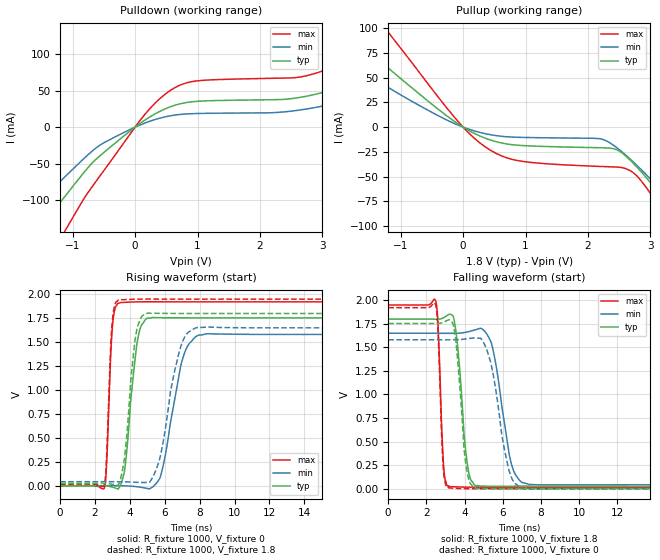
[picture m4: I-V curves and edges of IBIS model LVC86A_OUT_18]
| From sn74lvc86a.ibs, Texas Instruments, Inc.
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[Model]   LVC86A_OUT_18
Model_type  Output
Vref =   0
Rref =   1000
Cref =   30p
Vmeas =   0.9
| variable   typ   min   max
C_comp   6.28pF   4.38pF   8.30pF
| C_pullup   5.89pF   4.38pF   6.79pF
| C_pulldown   6.66pF   4.69pF   8.30pF
[Temperature Range]   40   100   -40
| Ambient temperature   25   85   -40
[Voltage range]   1.8   1.65   1.95
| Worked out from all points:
|   slope of the pulldown table from 0 to 0.27 V, typ, clamps not added: 17.1 ohm
|   slope of the pullup table from 0 to 0.27 V, typ, clamps not added: 29.9 ohm
|   rising waveform, R_fixture 1000, V_fixture 0: 20-80 % time 535ps typ, 904ps min, 249ps max; typ from 0 V to 1.75 V
|   falling waveform, R_fixture 1000, V_fixture 1.8: 20-80 % time 403ps typ, 707ps min, 210ps max; typ from 1.8 V to 0.027 V
|   rising waveform, R_fixture 1000, V_fixture 1.8: 20-80 % time 501ps typ, 925ps min, 244ps max; typ from 0.027 V to 1.8 V
|   falling waveform, R_fixture 1000, V_fixture 0: 20-80 % time 391ps typ, 743ps min, 203ps max; typ from 1.75 V to 0 V
[Pulldown]
| LVC86A_OUT_18
|   Voltage   I(typ)   I(min)   I(max)
-5.5V     -559.1mA   -452.2mA   -710.9mA
-2.18V    -208.5mA   -158.8mA   -285.4mA
-1.865V   -175.2mA   -131.6mA   -244.5mA
-1.48V    -133.9mA   -98.56mA   -193.1mA
-1.07V    -89.31mA   -63.76mA   -134.9mA
70mV      4.491mA    2.617mA    8.125mA
615mV     29.45mA    16.27mA    53.12mA
2.815V    43.69mA    25.92mA    72.1mA
4.325V    93.52mA    64.21mA    142.7mA
5.155V    134.5mA    96.03mA    199.6mA
6.155V    191.3mA    141.3mA    276.1mA
11V       510.2mA    405.2mA    689.3mA
[Pullup]
| LVC86A_OUT_18
|   Voltage   I(typ)   I(min)   I(max)
-5.5V     324.9mA    249.5mA    454.8mA
-2.68V    143.9mA    103mA      216.3mA
-2.015V   104.9mA    73.15mA    161.8mA
-1.32V    66.21mA    44.72mA    105.6mA
360mV     -11.3mA    -6.711mA   -20.18mA
985mV     -18.72mA   -10.42mA   -34.9mA
2.465V    -23.02mA   -20.97mA   -40.36mA
2.785V    -40.46mA   -38.76mA   -49.43mA
3.365V    -85.63mA   -77.45mA   -103.2mA
3.56V     -102.6mA   -91.66mA   -124.4mA
3.775V    -122mA     -107.8mA   -148.7mA
11V       -874.4mA   -739.7mA   -1.068A
[Ramp]
| LVC86A_OUT_18
| variable   typ   min   max
dV/dt_r   1.07/5.81E-10   0.97/9.92E-10   1.17/2.64E-10
dV/dt_f   1.10/4.49E-10   1.00/7.86E-10   1.20/2.28E-10
R_load = 1000
[Rising Waveform]
| LVC86A_OUT_18
R_fixture =   1000
C_fixture =   0
L_fixture =   0
V_fixture =   0
V_fixture_min = 0
V_fixture_max = 0
|   Time   V(typ)   V(min)   V(max)
0s        194.2pV    4.892nV    16.26pV
2.545ns   -67.28uV   692.4uV    -17.05mV
2.98ns    -12.92mV   538.6uV    1.618V
3.335ns   -33.35mV   301.3uV    1.908V
3.715ns   189mV      -781.9uV   1.917V
4.42ns    1.503V     -10.43mV   1.921V
4.985ns   1.75V      -27.87mV   1.922V
5.72ns    1.756V     78.66mV    1.922V
7.89ns    1.754V     1.57V      1.922V
24.99ns   1.754V     1.581V     1.922V
[Falling Waveform]
| LVC86A_OUT_18
R_fixture =   1000
C_fixture =   0
L_fixture =   0
V_fixture =   1.8
V_fixture_min = 1.65
V_fixture_max = 1.95
|   Time   V(typ)   V(min)   V(max)
0s        1.8V       1.65V      1.95V
2.5ns     1.799V     1.65V      1.986V
2.9ns     1.815V     1.649V     253.6mV
3.12ns    1.843V     1.649V     26.64mV
3.5ns     1.74V      1.649V     20.29mV
4.115ns   309.9mV    1.663V     16.51mV
4.58ns    32.42mV    1.687V     15.97mV
5.4ns     26.52mV    1.552V     16.02mV
7.035ns   26.87mV    63.93mV    16.27mV
24.99ns   27.13mV    42.42mV    16.27mV
[Rising Waveform]
| LVC86A_OUT_18
R_fixture =   1000
C_fixture =   0
L_fixture =   0
V_fixture =   1.8
V_fixture_min = 1.65
V_fixture_max = 1.95
|   Time   V(typ)   V(min)   V(max)
0s        27.13mV    42.42mV    16.27mV
2.53ns    26.95mV    42.98mV    7.892mV
2.965ns   16.64mV    42.56mV    1.659V
3.335ns   8.25mV     42.13mV    1.939V
4.33ns    1.562V     36.49mV    1.95V
4.955ns   1.799V     34.68mV    1.951V
5.72ns    1.801V     288.7mV    1.95V
6.92ns    1.8V       1.456V     1.95V
7.755ns   1.8V       1.648V     1.95V
24.99ns   1.8V       1.65V      1.95V
[Falling Waveform]
| LVC86A_OUT_18
R_fixture =   1000
C_fixture =   0
L_fixture =   0
V_fixture =   0
V_fixture_min = 0
V_fixture_max = 0
|   Time   V(typ)   V(min)   V(max)
0s        1.754V     1.581V     1.922V
2.485ns   1.753V     1.581V     1.949V
2.88ns    1.766V     1.58V      234.8mV
3.165ns   1.792V     1.58V      8.49mV
3.53ns    1.59V      1.581V     3.298mV
4.095ns   225.4mV    1.591V     80.75uV
4.515ns   7.983mV    1.599V     -355.5uV
5.255ns   -40.2uV    1.42V      -286.3uV
6.985ns   -239.4uV   4.098mV    -986.2nV
24.99ns   6.439nV    -207.2nV   24.14nV
